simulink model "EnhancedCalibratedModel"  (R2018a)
settings: Solver=VariableStepAuto  StartTime=0.0  StopTime=Sim_time  RelTol=1e-3
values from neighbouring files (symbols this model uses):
  Amplitude_Signal = 5    [ParameterInitializationFileFinal.m]
  Anglog_Input_Max = 3    [ParameterInitializationFileFinal.m]    (also in Panda_BEVintage_VPE_S_Data_CodeGen_Model.m = 10; Panda_BEVintage_VPE_S_Data_Enhanced_Model.m = 10)
  Anglog_Input_Min = 0    [ParameterInitializationFileFinal.m]    (also in Panda_BEVintage_VPE_S_Data_CodeGen_Model.m = -10; Panda_BEVintage_VPE_S_Data_Enhanced_Model.m = -10)
  Bias_Signal = 0    [ParameterInitializationFileFinal.m]
  Bits = 12    [ParameterInitializationFileFinal.m]    (also in Panda_BEVintage_VPE_S_Data_CodeGen_Model.m = 16; Panda_BEVintage_VPE_S_Data_Enhanced_Model.m = 16)
  CutOff_Freq = Frequency_Signal*8    (= 4)    [ParameterInitializationFileFinal.m]
  Digital_Output = 3.3    [ParameterInitializationFileFinal.m]
  fclk = 10e4    (= 100000)    [ParameterInitializationFileFinal.m]
  fpwm = fclk/2^BitsPWM    (= 24.4140625)    [ParameterInitializationFileFinal.m]
  Frequency_Signal = 1/2    (= 0.5)    [ParameterInitializationFileFinal.m]
  Full_Scale_Reading = Anglog_Input_Max-Anglog_Input_Min    (= 3)    [ParameterInitializationFileFinal.m]    (also in Panda_BEVintage_VPE_S_Data_CodeGen_Model.m = 20; Panda_BEVintage_VPE_S_Data_Enhanced_Model.m = 20)
  Max_Signal = Amplitude_Signal+Bias_Signal    (= 5)    [ParameterInitializationFileFinal.m]
  Min_Signal = -Amplitude_Signal+Bias_Signal    (= -5)    [ParameterInitializationFileFinal.m]
  Sampling_Time = 0.01    [ParameterInitializationFileFinal.m]    (also in Panda_BEVintage_VPE_S_Data_CodeGen_Model.m = 0.0001; Panda_BEVintage_VPE_S_Data_Enhanced_Model.m = 0.0001)
libraries: dspfdesign x2, pePwmGenerator x1

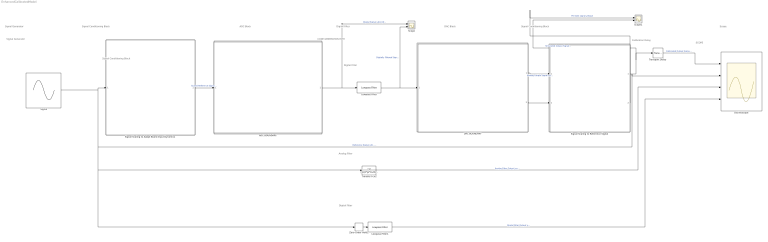
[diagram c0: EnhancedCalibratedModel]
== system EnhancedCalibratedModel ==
  note: Calibration Delay
  note: Signal Conditioning Block
  note: Signal Conditioning Block
  note: CODE GENERATION PART
  note: SCOPE
  note: Analog Filter
  note: Signal Generator
  note: Digital Filter
  note: Digital Filter
  note: ADC Block
  note: Signal Generator
  note: Digital Filter
  note: DAC Block
  note: Signal Conditioning Block
  note: Scope
  ADC BOUNDARY : Subsystem
  DAC BOUNDARY : Subsystem
  Lowpass Filter : dspfdesign/Lowpass Filter  FilterType=IIR  DesignForMinimumOrder=off  FilterOrder=1  PassbandFrequency=Frequency_Signal*4  StopbandFrequency=1  PassbandRipple=1  StopbandAttenuation=80  InheritSampleRate=on  SampleRate=Frequency_Signal*5  SimulateUsing=Interpreted execution  roundingMode=Floor  coeffsDataTypeStr=fixdt(1,16)
  Lowpass Filter1 : dspfdesign/Lowpass Filter  FilterType=IIR  DesignForMinimumOrder=off  FilterOrder=1  PassbandFrequency=Frequency_Signal*4  StopbandFrequency=1  PassbandRipple=1  StopbandAttenuation=80  InheritSampleRate=on  SampleRate=Frequency_Signal/4  SimulateUsing=Interpreted execution  roundingMode=Floor  coeffsDataTypeStr=fixdt(1,16)
  Oscillioscope : Scope  NumInputPorts=4
  Scope : Scope  NumInputPorts=2
  Scope1 : Scope  NumInputPorts=2
  Signal : Sin  Amplitude=Amplitude_Signal  Bias=Bias_Signal  Frequency=2*pi*Frequency_Signal  SampleTime=0
  Signal Scaling to Adapt Board Input Dynamics : Subsystem
  Signal Scaling to Reference Signal : Subsystem
  Transfer Fcn2 : TransferFcn  Denominator=[1/(2*pi*CutOff_Freq) 1]
  Transport Delay : TransportDelay  DelayTime=0.023
  Zero-Order Hold2 : ZeroOrderHold  SampleTime=Sampling_Time
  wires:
  Signal/1 -> Signal Scaling to Adapt Board Input Dynamics/1(Reference Signal u(t)), Oscillioscope/2, Zero-Order Hold2/1, Transfer Fcn2/1  "Reference Signal u(t) -5 To 5 [v]  1/2 [Hz]"
  Transfer Fcn2/1 -> Oscillioscope/3  "Analog Filter Output ya(t)"
  Signal Scaling to Adapt Board Input Dynamics/1(Scaled Reference Signal us(t)) -> ADC BOUNDARY/1(Scaled Reference Signal)  "Scaled Reference Signal us(t)"
  Signal Scaling to Reference Signal/1(Simulated Output Signal y(t) [-5 To 5] [V]) -> Scope1/2, Transport Delay/1  "Simulated Output Signal y(t)"
  ADC BOUNDARY/1("Digital Signal ud(z) [0-4095] 12 bits Sampling Time 0.01s ") -> Scope/1, Lowpass Filter/1  "Digital Signal ud(z) [0-4095] 12 bits  Sampling Time 0.01s"
  Lowpass Filter/1 -> Scope/2, DAC BOUNDARY/1("Digital Signal ud(z) [0-4095] 12 bits Sampling Time 0.01s  ")  "Digitally Filtered Signal udf(z) [0-4095] 12 bits  Sampling Time 0.01s"
  DAC BOUNDARY/1(Analog Output Signal ya(t) [0-3.3] [V]) -> Signal Scaling to Reference Signal/1(Analog Output Signal ya(t) [0-3.3] [V])  "Analog Output Signal ya(t) [0-3.3] [V]"
  Lowpass Filter1/1 -> Oscillioscope/4  "Digital Filter Output yD(t)"
  Zero-Order Hold2/1 -> Lowpass Filter1/1
  Signal Scaling to Reference Signal/2(Scaled Filtered Digital Output (Before PWM block) ydss(z) [-5 To 5] [V]) -> Scope1/1  "Pre-DAC signal ydss(z)"
  DAC BOUNDARY/2(Scaled Filtered Digital Output yds(z) [0-3] [V]) -> Signal Scaling to Reference Signal/2(Scaled Filtered Digital Output yds(z) [0-3] [V])
  Transport Delay/1 -> Oscillioscope/1  "Calibrated Output Signal yy(t)"

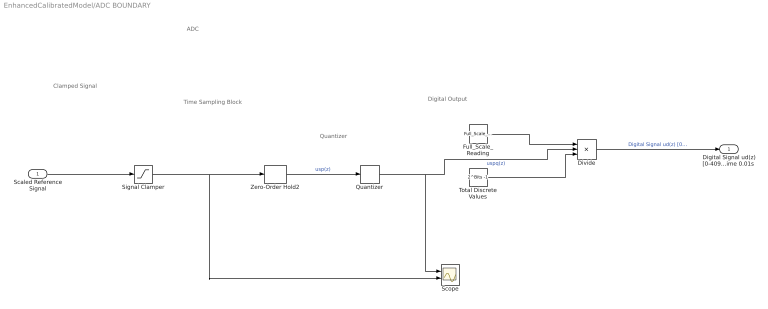
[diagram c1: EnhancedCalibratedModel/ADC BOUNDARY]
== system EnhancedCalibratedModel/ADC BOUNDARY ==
  note: Quantizer
  note: Time Sampling Block
  note: Digital Output
  note: Clamped Signal
  note: ADC
  Scaled Reference Signal : Inport
  Divide : Product  Inputs=/**
  Full_Scale_Reading : Constant  Value=Full_Scale_Reading
  Quantizer : Quantizer  QuantizationInterval=Full_Scale_Reading/(2^Bits-1 )
  Scope : Scope  NumInputPorts=2
  Signal Clamper : Saturate  UpperLimit=Anglog_Input_Max  LowerLimit=0
  Total Discrete Values : Constant  Value=2^Bits -1
  Zero-Order Hold2 : ZeroOrderHold  SampleTime=Sampling_Time
  "Digital Signal ud(z) [0-4095] 12 bits Sampling Time 0.01s " : Outport
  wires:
  Signal Clamper/1 -> Scope/2, Zero-Order Hold2/1
  Scaled Reference Signal/1 -> Signal Clamper/1
  Full_Scale_Reading/1 -> Divide/1
  Total Discrete Values/1 -> Divide/3
  Quantizer/1 -> Scope/1, Divide/2  "uspq(z)"
  Divide/1 -> "Digital Signal ud(z) [0-4095] 12 bits Sampling Time 0.01s "/1  "Digital Signal ud(z) [0-4095] 12 bits  Sampling Time 0.01s"
  Zero-Order Hold2/1 -> Quantizer/1  "usp(z)"

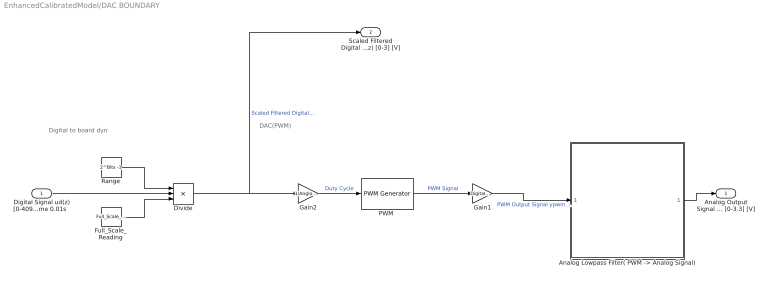
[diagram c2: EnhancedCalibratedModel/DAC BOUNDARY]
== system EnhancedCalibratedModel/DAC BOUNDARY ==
  note: DAC(PWM)
  note: Digital to board dyn
  "Digital Signal ud(z) [0-4095] 12 bits Sampling Time 0.01s  " : Inport
  "Analog Lowpass Filter( PWM -> Analog Signal)" : Subsystem
  Divide : Product  Inputs=/**
  Full_Scale_Reading : Constant  Value=Full_Scale_Reading
  Gain1 : Gain  Gain=Digital_Output
  Gain2 : Gain  Gain=1/Anglog_Input_Max
  "PWM " : pePwmGenerator/PWM Generator  CarrCount=Up  Tper=1/fpwm  Ts=1/fclk
  Range : Constant  Value=2^Bits -1
  Analog Output Signal ya(t) [0-3.3] [V] : Outport
  Scaled Filtered Digital Output yds(z) [0-3] [V] : Outport  Port=2
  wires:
  Gain2/1 -> "PWM "/1  "Duty Cycle"
  "PWM "/1 -> Gain1/1  "PWM Signal"
  Gain1/1 -> "Analog Lowpass Filter( PWM -> Analog Signal)"/1("PWM  Signal ")  "PWM Output Signal ypwm \t\t[0-1]"
  Range/1 -> Divide/1
  Full_Scale_Reading/1 -> Divide/3
  "Digital Signal ud(z) [0-4095] 12 bits Sampling Time 0.01s  "/1 -> Divide/2
  Divide/1 -> Scaled Filtered Digital Output yds(z) [0-3] [V]/1, Gain2/1  "Scaled Filtered Digital Output yds(z) \t\t\t[0-3] \t\t\t [V]"
  "Analog Lowpass Filter( PWM -> Analog Signal)"/1(ya(t)) -> Analog Output Signal ya(t) [0-3.3] [V]/1

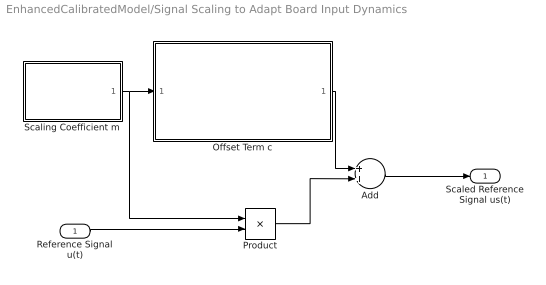
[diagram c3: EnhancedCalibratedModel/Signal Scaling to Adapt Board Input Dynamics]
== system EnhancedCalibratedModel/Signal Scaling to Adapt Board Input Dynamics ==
  Reference Signal u(t) : Inport
  Add : Sum
  Offset Term c : Subsystem
  Product : Product
  Scaling Coefficient m : Subsystem
  Scaled Reference Signal us(t) : Outport
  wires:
  Scaling Coefficient m/1(Scaling Coefficient m) -> Product/1, Offset Term c/1(Scaling Coefficent m)
  Reference Signal u(t)/1 -> Product/2
  Product/1 -> Add/2
  Offset Term c/1("Offset Term c ") -> Add/1
  Add/1 -> Scaled Reference Signal us(t)/1

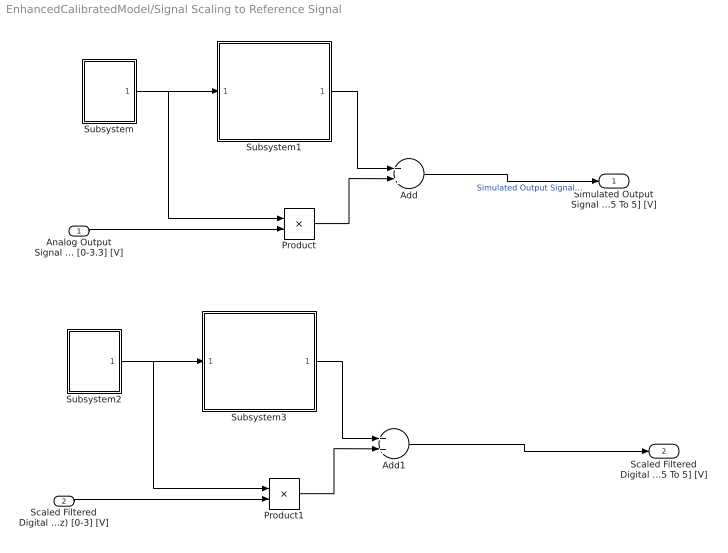
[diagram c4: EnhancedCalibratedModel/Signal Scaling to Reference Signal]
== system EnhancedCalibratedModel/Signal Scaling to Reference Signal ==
  Analog Output Signal ya(t) [0-3.3] [V] : Inport
  Scaled Filtered Digital Output yds(z) [0-3] [V] : Inport  Port=2
  Add : Sum
  Add1 : Sum
  Product : Product
  Product1 : Product
  Subsystem : Subsystem
  Subsystem1 : Subsystem
  Subsystem2 : Subsystem
  Subsystem3 : Subsystem
  Simulated Output Signal y(t) [-5 To 5] [V] : Outport
  Scaled Filtered Digital Output (Before PWM block) ydss(z) [-5 To 5] [V] : Outport  Port=2
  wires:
  Product/1 -> Add/2
  Add/1 -> Simulated Output Signal y(t) [-5 To 5] [V]/1  "Simulated Output Signal y(t) \t\t[-5 To 5] \t\t     [V]"
  Subsystem/1("Gradient ") -> Product/1, Subsystem1/1("Gradient ")
  Subsystem1/1("Offset ") -> Add/1
  Analog Output Signal ya(t) [0-3.3] [V]/1 -> Product/2
  Product1/1 -> Add1/2
  Subsystem3/1("Offset ") -> Add1/1
  Scaled Filtered Digital Output yds(z) [0-3] [V]/1 -> Product1/2
  Subsystem2/1("Gradient ") -> Product1/1, Subsystem3/1("Gradient ")
  Add1/1 -> Scaled Filtered Digital Output (Before PWM block) ydss(z) [-5 To 5] [V]/1

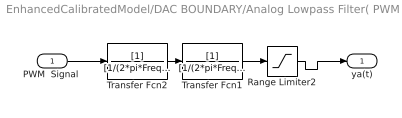
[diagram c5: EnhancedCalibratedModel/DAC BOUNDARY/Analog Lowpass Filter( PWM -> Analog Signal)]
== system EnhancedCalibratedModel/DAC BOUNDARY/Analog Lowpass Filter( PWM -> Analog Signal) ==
  "PWM  Signal " : Inport
  Range Limiter2 : Saturate  UpperLimit=Digital_Output  LowerLimit=0
  Transfer Fcn1 : TransferFcn  Denominator=[1/(2*pi*Frequency_Signal*5) 1]
  Transfer Fcn2 : TransferFcn  Denominator=[1/(2*pi*Frequency_Signal*5) 1]
  ya(t) : Outport
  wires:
  Range Limiter2/1 -> ya(t)/1
  "PWM  Signal "/1 -> Transfer Fcn2/1
  Transfer Fcn2/1 -> Transfer Fcn1/1
  Transfer Fcn1/1 -> Range Limiter2/1

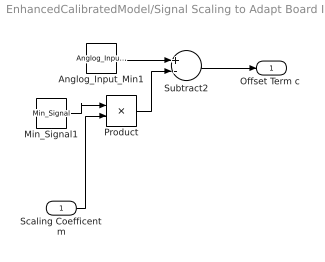
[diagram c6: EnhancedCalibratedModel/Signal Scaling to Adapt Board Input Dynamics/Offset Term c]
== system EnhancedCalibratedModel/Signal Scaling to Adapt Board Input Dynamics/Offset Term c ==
  Scaling Coefficent m : Inport
  Anglog_Input_Min1 : Constant  Value=Anglog_Input_Min
  Min_Signal1 : Constant  Value=Min_Signal
  Product : Product
  Subtract2 : Sum  Inputs=+-
  "Offset Term c " : Outport
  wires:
  Min_Signal1/1 -> Product/1
  Scaling Coefficent m/1 -> Product/2
  Product/1 -> Subtract2/2
  Subtract2/1 -> "Offset Term c "/1
  Anglog_Input_Min1/1 -> Subtract2/1

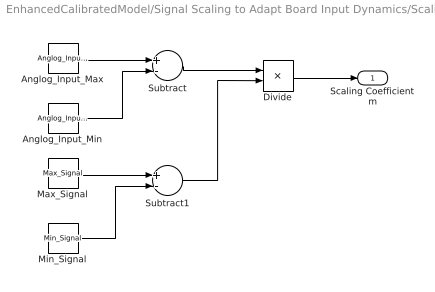
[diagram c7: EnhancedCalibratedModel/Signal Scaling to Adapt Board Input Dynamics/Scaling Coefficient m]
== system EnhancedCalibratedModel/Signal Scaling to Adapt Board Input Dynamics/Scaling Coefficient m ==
  Anglog_Input_Max : Constant  Value=Anglog_Input_Max
  Anglog_Input_Min : Constant  Value=Anglog_Input_Min
  Divide : Product  Inputs=*/
  Max_Signal : Constant  Value=Max_Signal
  Min_Signal : Constant  Value=Min_Signal
  Subtract : Sum  Inputs=+-
  Subtract1 : Sum  Inputs=+-
  Scaling Coefficient m : Outport
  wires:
  Divide/1 -> Scaling Coefficient m/1
  Subtract1/1 -> Divide/2
  Subtract/1 -> Divide/1
  Anglog_Input_Min/1 -> Subtract/2
  Min_Signal/1 -> Subtract1/2
  Max_Signal/1 -> Subtract1/1
  Anglog_Input_Max/1 -> Subtract/1

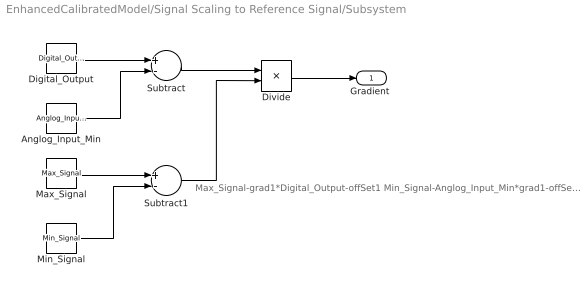
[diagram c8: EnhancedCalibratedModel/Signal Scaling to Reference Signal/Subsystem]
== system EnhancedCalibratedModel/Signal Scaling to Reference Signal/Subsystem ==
  note: Max_Signal-grad1*Digital_Output-offSet1 Min_Signal-Anglog_Input_Min*grad1-offSet1
  Anglog_Input_Min : Constant  Value=Anglog_Input_Min
  Digital_Output : Constant  Value=Digital_Output
  Divide : Product  Inputs=/*
  Max_Signal : Constant  Value=Max_Signal
  Min_Signal : Constant  Value=Min_Signal
  Subtract : Sum  Inputs=+-
  Subtract1 : Sum  Inputs=+-
  "Gradient " : Outport
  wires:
  Divide/1 -> "Gradient "/1
  Subtract1/1 -> Divide/2
  Subtract/1 -> Divide/1
  Anglog_Input_Min/1 -> Subtract/2
  Min_Signal/1 -> Subtract1/2
  Max_Signal/1 -> Subtract1/1
  Digital_Output/1 -> Subtract/1

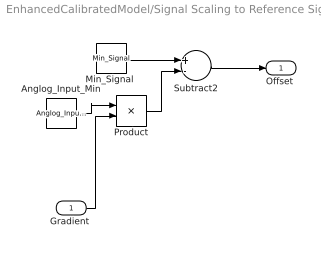
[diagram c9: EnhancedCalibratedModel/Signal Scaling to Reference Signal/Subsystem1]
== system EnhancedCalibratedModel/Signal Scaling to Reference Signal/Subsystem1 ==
  "Gradient " : Inport
  Anglog_Input_Min : Constant  Value=Anglog_Input_Min
  "Min_Signal " : Constant  Value=Min_Signal
  Product : Product
  Subtract2 : Sum  Inputs=+-
  "Offset " : Outport
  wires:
  Anglog_Input_Min/1 -> Product/1
  "Gradient "/1 -> Product/2
  Product/1 -> Subtract2/2
  Subtract2/1 -> "Offset "/1
  "Min_Signal "/1 -> Subtract2/1

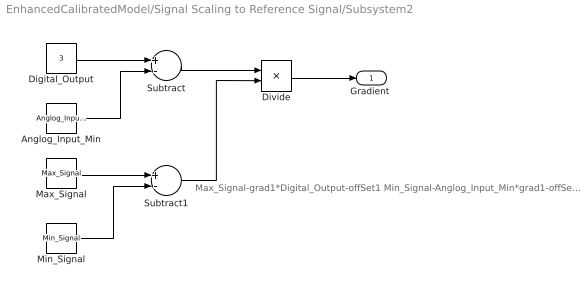
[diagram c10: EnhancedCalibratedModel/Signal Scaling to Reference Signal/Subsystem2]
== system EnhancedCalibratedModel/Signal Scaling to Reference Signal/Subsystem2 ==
  note: Max_Signal-grad1*Digital_Output-offSet1 Min_Signal-Anglog_Input_Min*grad1-offSet1
  Anglog_Input_Min : Constant  Value=Anglog_Input_Min
  Digital_Output : Constant  Value=3
  Divide : Product  Inputs=/*
  Max_Signal : Constant  Value=Max_Signal
  Min_Signal : Constant  Value=Min_Signal
  Subtract : Sum  Inputs=+-
  Subtract1 : Sum  Inputs=+-
  "Gradient " : Outport
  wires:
  Divide/1 -> "Gradient "/1
  Subtract1/1 -> Divide/2
  Subtract/1 -> Divide/1
  Anglog_Input_Min/1 -> Subtract/2
  Min_Signal/1 -> Subtract1/2
  Max_Signal/1 -> Subtract1/1
  Digital_Output/1 -> Subtract/1

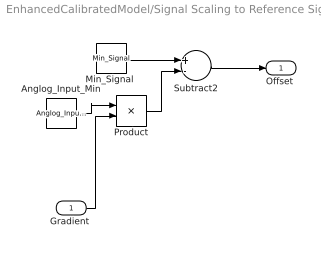
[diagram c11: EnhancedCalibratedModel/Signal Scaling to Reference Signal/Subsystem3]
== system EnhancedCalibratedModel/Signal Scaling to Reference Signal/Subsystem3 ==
  "Gradient " : Inport
  Anglog_Input_Min : Constant  Value=Anglog_Input_Min
  "Min_Signal " : Constant  Value=Min_Signal
  Product : Product
  Subtract2 : Sum  Inputs=+-
  "Offset " : Outport
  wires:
  Anglog_Input_Min/1 -> Product/1
  "Gradient "/1 -> Product/2
  Product/1 -> Subtract2/2
  Subtract2/1 -> "Offset "/1
  "Min_Signal "/1 -> Subtract2/1
